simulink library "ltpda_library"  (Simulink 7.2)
settings: Solver=ode45  SolverMode=SingleTasking  StartTime=0.0  StopTime=10.0  RelTol=1e-3
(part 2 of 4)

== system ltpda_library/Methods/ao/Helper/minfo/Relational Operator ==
  eq : Subsystem  Tag=method minfo  AncestorBlock=libraryBase/function
  ne : Subsystem  Tag=method minfo  AncestorBlock=libraryBase/function

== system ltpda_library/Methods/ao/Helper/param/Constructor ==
  param : Subsystem  Tag=method param  AncestorBlock=libraryBase/constructor

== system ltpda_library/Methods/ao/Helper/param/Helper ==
  isprop : Subsystem  Tag=method param  AncestorBlock=libraryBase/function
  mux : Subsystem  Tag=method param  AncestorBlock=libraryBase/function

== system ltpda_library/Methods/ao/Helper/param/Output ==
  char : Subsystem  Tag=method param  AncestorBlock=libraryBase/output
  display : Subsystem  Tag=method param  AncestorBlock=libraryBase/output
  string : Subsystem  Tag=method param  AncestorBlock=libraryBase/output

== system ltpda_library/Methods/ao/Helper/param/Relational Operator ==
  eq : Subsystem  Tag=method param  AncestorBlock=libraryBase/function
  ne : Subsystem  Tag=method param  AncestorBlock=libraryBase/function

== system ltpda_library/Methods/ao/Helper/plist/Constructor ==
  plist : Subsystem  Tag=method plist  AncestorBlock=libraryBase/constructor
  rebuild : Subsystem  Tag=method parfrac  AncestorBlock=libraryBase/constructor

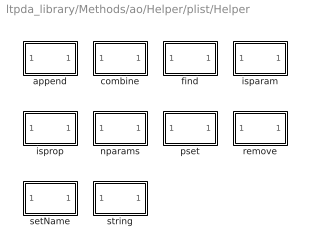
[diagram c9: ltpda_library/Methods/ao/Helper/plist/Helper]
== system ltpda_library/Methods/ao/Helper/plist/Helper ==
  append : Subsystem  Tag=method plist  AncestorBlock=libraryBase/function
  combine : Subsystem  Tag=method plist  AncestorBlock=libraryBase/function
  find : Subsystem  Tag=method plist  AncestorBlock=libraryBase/function
  isparam : Subsystem  Tag=method plist  AncestorBlock=libraryBase/function
  isprop : Subsystem  Tag=method plist  AncestorBlock=libraryBase/function
  nparams : Subsystem  Tag=method plist  AncestorBlock=libraryBase/function
  pset : Subsystem  Tag=method plist  AncestorBlock=libraryBase/function
  remove : Subsystem  Tag=method plist  AncestorBlock=libraryBase/function
  setName : Subsystem  Tag=method plist  AncestorBlock=libraryBase/function
  string : Subsystem  Tag=method plist  AncestorBlock=libraryBase/function

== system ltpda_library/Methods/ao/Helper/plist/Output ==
  char : Subsystem  Tag=method plist  AncestorBlock=libraryBase/output
  display : Subsystem  Tag=method plist  AncestorBlock=libraryBase/output
  save : Subsystem  Tag=method plist  AncestorBlock=libraryBase/output

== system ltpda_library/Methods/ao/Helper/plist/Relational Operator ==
  eq : Subsystem  Tag=method plist  AncestorBlock=libraryBase/function
  ne : Subsystem  Tag=method plist  AncestorBlock=libraryBase/function

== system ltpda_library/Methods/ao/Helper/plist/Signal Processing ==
  resp : Subsystem  Tag=method plist  AncestorBlock=libraryBase/function

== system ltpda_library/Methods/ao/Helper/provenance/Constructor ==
  provenance : Subsystem  Tag=method provenance  AncestorBlock=libraryBase/constructor

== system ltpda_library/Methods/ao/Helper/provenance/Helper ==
  isprop : Subsystem  Tag=method provenance  AncestorBlock=libraryBase/function

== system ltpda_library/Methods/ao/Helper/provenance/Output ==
  char : Subsystem  Tag=method provenance  AncestorBlock=libraryBase/output
  display : Subsystem  Tag=method provenance  AncestorBlock=libraryBase/output
  string : Subsystem  Tag=method provenance  AncestorBlock=libraryBase/output

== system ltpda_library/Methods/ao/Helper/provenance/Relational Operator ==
  eq : Subsystem  Tag=method provenance  AncestorBlock=libraryBase/function
  ne : Subsystem  Tag=method provenance  AncestorBlock=libraryBase/function

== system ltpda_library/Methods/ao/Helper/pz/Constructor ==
  pz : Subsystem  Tag=method pz  AncestorBlock=libraryBase/constructor

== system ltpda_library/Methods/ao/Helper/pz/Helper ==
  isprop : Subsystem  Tag=method pz  AncestorBlock=libraryBase/function

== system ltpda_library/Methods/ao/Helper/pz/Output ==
  char : Subsystem  Tag=method pz  AncestorBlock=libraryBase/output
  display : Subsystem  Tag=method pz  AncestorBlock=libraryBase/output
  string : Subsystem  Tag=method pz  AncestorBlock=libraryBase/output

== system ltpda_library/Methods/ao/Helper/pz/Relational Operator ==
  eq : Subsystem  Tag=method pz  AncestorBlock=libraryBase/function
  ne : Subsystem  Tag=method pz  AncestorBlock=libraryBase/function

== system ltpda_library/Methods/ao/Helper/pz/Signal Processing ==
  resp : Subsystem  Tag=method pz  AncestorBlock=libraryBase/function

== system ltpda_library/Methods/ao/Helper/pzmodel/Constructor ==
  pzmodel : Subsystem  Tag=method pzmodel  AncestorBlock=libraryBase/constructor
  rebuild : Subsystem  Tag=method pzmodel  AncestorBlock=libraryBase/constructor

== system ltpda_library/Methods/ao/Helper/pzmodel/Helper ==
  isprop : Subsystem  Tag=method pzmodel  AncestorBlock=libraryBase/function
  setIunits : Subsystem  Tag=method pzmodel  AncestorBlock=libraryBase/function
  setName : Subsystem  Tag=method pzmodel  AncestorBlock=libraryBase/function
  setOunits : Subsystem  Tag=method pzmodel  AncestorBlock=libraryBase/function
  setProperties : Subsystem  Tag=method pzmodel  AncestorBlock=libraryBase/function
  string : Subsystem  Tag=method pzmodel  AncestorBlock=libraryBase/function

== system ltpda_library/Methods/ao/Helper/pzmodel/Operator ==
  tomfir : Subsystem  Tag=method pzmodel  AncestorBlock=libraryBase/function
  tomiir : Subsystem  Tag=method pzmodel  AncestorBlock=libraryBase/function

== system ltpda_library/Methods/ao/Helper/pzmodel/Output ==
  char : Subsystem  Tag=method pzmodel  AncestorBlock=libraryBase/output
  display : Subsystem  Tag=method pzmodel  AncestorBlock=libraryBase/output
  save : Subsystem  Tag=method pzmodel  AncestorBlock=libraryBase/output
  type : Subsystem  Tag=method pzmodel  AncestorBlock=libraryBase/output

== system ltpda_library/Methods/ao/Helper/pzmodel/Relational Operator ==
  eq : Subsystem  Tag=method pzmodel  AncestorBlock=libraryBase/function
  ne : Subsystem  Tag=method pzmodel  AncestorBlock=libraryBase/function

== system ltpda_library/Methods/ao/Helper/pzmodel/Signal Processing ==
  fngen : Subsystem  Tag=method pzmodel  AncestorBlock=libraryBase/function
  resp : Subsystem  Tag=method pzmodel  AncestorBlock=libraryBase/function

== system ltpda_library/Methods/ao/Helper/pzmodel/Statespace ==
  report : Subsystem  Tag=method pzmodel  AncestorBlock=libraryBase/function

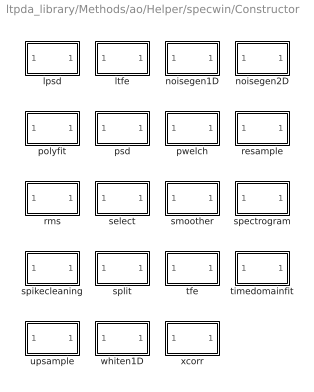
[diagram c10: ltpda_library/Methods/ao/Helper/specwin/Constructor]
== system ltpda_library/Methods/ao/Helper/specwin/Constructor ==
  lpsd : Subsystem  Tag=method specwin  AncestorBlock=libraryBase/constructor  Tag=method ao  AncestorBlock=libraryBase/function
  ltfe : Subsystem  Tag=method ao  AncestorBlock=libraryBase/function
  noisegen1D : Subsystem  Tag=method ao  AncestorBlock=libraryBase/function
  noisegen2D : Subsystem  Tag=method ao  AncestorBlock=libraryBase/function
  polyfit : Subsystem  Tag=method ao  AncestorBlock=libraryBase/function
  psd : Subsystem  Tag=method ao  AncestorBlock=libraryBase/function
  pwelch : Subsystem  Tag=method ao  AncestorBlock=libraryBase/function
  resample : Subsystem  Tag=method ao  AncestorBlock=libraryBase/function
  rms : Subsystem  Tag=method ao  AncestorBlock=libraryBase/function
  select : Subsystem  Tag=method ao  AncestorBlock=libraryBase/function
  smoother : Subsystem  Tag=method ao  AncestorBlock=libraryBase/function
  spectrogram : Subsystem  Tag=method ao  AncestorBlock=libraryBase/function
  spikecleaning : Subsystem  Tag=method ao  AncestorBlock=libraryBase/function
  split : Subsystem  Tag=method ao  AncestorBlock=libraryBase/function
  tfe : Subsystem  Tag=method ao  AncestorBlock=libraryBase/function
  timedomainfit : Subsystem  Tag=method ao  AncestorBlock=libraryBase/function
  upsample : Subsystem  Tag=method ao  AncestorBlock=libraryBase/function
  whiten1D : Subsystem  Tag=method ao  AncestorBlock=libraryBase/function
  xcorr : Subsystem  Tag=method ao  AncestorBlock=libraryBase/function

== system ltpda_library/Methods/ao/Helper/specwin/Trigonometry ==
  acos : Subsystem  Tag=method ao  AncestorBlock=libraryBase/function
  asin : Subsystem  Tag=method ao  AncestorBlock=libraryBase/function
  atan : Subsystem  Tag=method ao  AncestorBlock=libraryBase/function
  atan2 : Subsystem  Tag=method ao  AncestorBlock=libraryBase/function
  cos : Subsystem  Tag=method ao  AncestorBlock=libraryBase/function
  sin : Subsystem  Tag=method ao  AncestorBlock=libraryBase/function
  tan : Subsystem  Tag=method ao  AncestorBlock=libraryBase/function

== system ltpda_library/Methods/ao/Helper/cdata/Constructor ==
  cdata : Subsystem  Tag=method cdata  AncestorBlock=libraryBase/constructor

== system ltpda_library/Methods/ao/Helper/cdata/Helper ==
  isprop : Subsystem  Tag=method cdata  AncestorBlock=libraryBase/function

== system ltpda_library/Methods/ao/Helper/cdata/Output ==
  display : Subsystem  Tag=method cdata  AncestorBlock=libraryBase/output

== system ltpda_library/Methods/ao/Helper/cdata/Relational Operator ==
  eq : Subsystem  Tag=method cdata  AncestorBlock=libraryBase/function
  ne : Subsystem  Tag=method cdata  AncestorBlock=libraryBase/function

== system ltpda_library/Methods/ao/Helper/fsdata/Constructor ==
  fsdata : Subsystem  Tag=method fsdata  AncestorBlock=libraryBase/constructor

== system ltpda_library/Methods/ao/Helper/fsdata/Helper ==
  isprop : Subsystem  Tag=method fsdata  AncestorBlock=libraryBase/function

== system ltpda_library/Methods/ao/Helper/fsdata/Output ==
  char : Subsystem  Tag=method fsdata  AncestorBlock=libraryBase/output
  display : Subsystem  Tag=method fsdata  AncestorBlock=libraryBase/output

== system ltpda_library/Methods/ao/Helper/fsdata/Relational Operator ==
  eq : Subsystem  Tag=method fsdata  AncestorBlock=libraryBase/function
  ne : Subsystem  Tag=method fsdata  AncestorBlock=libraryBase/function

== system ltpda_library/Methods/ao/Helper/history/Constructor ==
  history : Subsystem  Tag=method history  AncestorBlock=libraryBase/constructor
  rebuild : Subsystem  Tag=method history  AncestorBlock=libraryBase/constructor

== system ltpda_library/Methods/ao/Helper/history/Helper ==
  isprop : Subsystem  Tag=method history  AncestorBlock=libraryBase/function

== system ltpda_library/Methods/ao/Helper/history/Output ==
  char : Subsystem  Tag=method history  AncestorBlock=libraryBase/output
  display : Subsystem  Tag=method history  AncestorBlock=libraryBase/output
  dotview : Subsystem  Tag=method history  AncestorBlock=libraryBase/output
  hist2dot : Subsystem  Tag=method history  AncestorBlock=libraryBase/output
  hist2m : Subsystem  Tag=method history  AncestorBlock=libraryBase/output
  plot : Subsystem  Tag=method history  AncestorBlock=libraryBase/output
  string : Subsystem  Tag=method history  AncestorBlock=libraryBase/output

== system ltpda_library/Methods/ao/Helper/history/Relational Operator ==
  eq : Subsystem  Tag=method history  AncestorBlock=libraryBase/function
  ne : Subsystem  Tag=method history  AncestorBlock=libraryBase/function

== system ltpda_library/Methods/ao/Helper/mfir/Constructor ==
  mfir : Subsystem  Tag=method mfir  AncestorBlock=libraryBase/constructor
  rebuild : Subsystem  Tag=method mfir  AncestorBlock=libraryBase/constructor

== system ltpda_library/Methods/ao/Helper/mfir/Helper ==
  isprop : Subsystem  Tag=method mfir  AncestorBlock=libraryBase/function
  redesign : Subsystem  Tag=method mfir  AncestorBlock=libraryBase/function
  setIunits : Subsystem  Tag=method mfir  AncestorBlock=libraryBase/function
  setName : Subsystem  Tag=method mfir  AncestorBlock=libraryBase/function
  setOunits : Subsystem  Tag=method mfir  AncestorBlock=libraryBase/function
  setProperties : Subsystem  Tag=method mfir  AncestorBlock=libraryBase/function

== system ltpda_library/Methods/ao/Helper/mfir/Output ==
  char : Subsystem  Tag=method mfir  AncestorBlock=libraryBase/output
  display : Subsystem  Tag=method mfir  AncestorBlock=libraryBase/output
  report : Subsystem  Tag=method mfir  AncestorBlock=libraryBase/output
  save : Subsystem  Tag=method mfir  AncestorBlock=libraryBase/output
  string : Subsystem  Tag=method mfir  AncestorBlock=libraryBase/output
  type : Subsystem  Tag=method mfir  AncestorBlock=libraryBase/output

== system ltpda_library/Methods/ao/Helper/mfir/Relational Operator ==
  eq : Subsystem  Tag=method mfir  AncestorBlock=libraryBase/function
  ne : Subsystem  Tag=method mfir  AncestorBlock=libraryBase/function

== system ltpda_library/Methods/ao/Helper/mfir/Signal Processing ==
  oldresp : Subsystem  Tag=method mfir  AncestorBlock=libraryBase/function
  resp : Subsystem  Tag=method mfir  AncestorBlock=libraryBase/function

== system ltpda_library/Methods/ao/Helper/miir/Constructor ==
  miir : Subsystem  Tag=method miir  AncestorBlock=libraryBase/constructor
  rebuild : Subsystem  Tag=method miir  AncestorBlock=libraryBase/constructor

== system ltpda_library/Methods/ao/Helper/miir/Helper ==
  isprop : Subsystem  Tag=method miir  AncestorBlock=libraryBase/function
  redesign : Subsystem  Tag=method miir  AncestorBlock=libraryBase/function
  setIunits : Subsystem  Tag=method miir  AncestorBlock=libraryBase/function
  setName : Subsystem  Tag=method miir  AncestorBlock=libraryBase/function
  setOunits : Subsystem  Tag=method miir  AncestorBlock=libraryBase/function
  setProperties : Subsystem  Tag=method miir  AncestorBlock=libraryBase/function

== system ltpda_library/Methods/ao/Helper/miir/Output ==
  char : Subsystem  Tag=method miir  AncestorBlock=libraryBase/output
  display : Subsystem  Tag=method miir  AncestorBlock=libraryBase/output
  report : Subsystem  Tag=method miir  AncestorBlock=libraryBase/output
  save : Subsystem  Tag=method miir  AncestorBlock=libraryBase/output
  string : Subsystem  Tag=method miir  AncestorBlock=libraryBase/output
  type : Subsystem  Tag=method miir  AncestorBlock=libraryBase/output

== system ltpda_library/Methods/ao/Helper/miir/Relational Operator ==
  eq : Subsystem  Tag=method miir  AncestorBlock=libraryBase/function
  ne : Subsystem  Tag=method miir  AncestorBlock=libraryBase/function

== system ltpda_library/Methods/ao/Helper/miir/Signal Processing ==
  oldresp : Subsystem  Tag=method miir  AncestorBlock=libraryBase/function
  resp : Subsystem  Tag=method miir  AncestorBlock=libraryBase/function

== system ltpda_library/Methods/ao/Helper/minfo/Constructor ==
  minfo : Subsystem  Tag=method minfo  AncestorBlock=libraryBase/constructor

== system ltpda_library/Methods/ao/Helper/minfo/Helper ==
  isprop : Subsystem  Tag=method minfo  AncestorBlock=libraryBase/function

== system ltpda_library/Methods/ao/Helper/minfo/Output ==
  char : Subsystem  Tag=method minfo  AncestorBlock=libraryBase/output
  display : Subsystem  Tag=method minfo  AncestorBlock=libraryBase/output

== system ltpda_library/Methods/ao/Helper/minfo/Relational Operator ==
  eq : Subsystem  Tag=method minfo  AncestorBlock=libraryBase/function
  ne : Subsystem  Tag=method minfo  AncestorBlock=libraryBase/function

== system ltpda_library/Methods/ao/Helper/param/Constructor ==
  param : Subsystem  Tag=method param  AncestorBlock=libraryBase/constructor

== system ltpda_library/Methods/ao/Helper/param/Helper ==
  isprop : Subsystem  Tag=method param  AncestorBlock=libraryBase/function
  mux : Subsystem  Tag=method param  AncestorBlock=libraryBase/function

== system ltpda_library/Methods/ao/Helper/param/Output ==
  char : Subsystem  Tag=method param  AncestorBlock=libraryBase/output
  display : Subsystem  Tag=method param  AncestorBlock=libraryBase/output
  string : Subsystem  Tag=method param  AncestorBlock=libraryBase/output

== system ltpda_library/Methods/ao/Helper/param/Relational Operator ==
  eq : Subsystem  Tag=method param  AncestorBlock=libraryBase/function
  ne : Subsystem  Tag=method param  AncestorBlock=libraryBase/function

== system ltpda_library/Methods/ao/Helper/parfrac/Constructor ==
  parfrac : Subsystem  Tag=method parfrac  AncestorBlock=libraryBase/constructor
  rebuild : Subsystem  Tag=method parfrac  AncestorBlock=libraryBase/constructor

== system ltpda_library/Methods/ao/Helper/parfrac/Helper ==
  isprop : Subsystem  Tag=method parfrac  AncestorBlock=libraryBase/function
  setIunits : Subsystem  Tag=method parfrac  AncestorBlock=libraryBase/function
  setName : Subsystem  Tag=method parfrac  AncestorBlock=libraryBase/function
  setOunits : Subsystem  Tag=method parfrac  AncestorBlock=libraryBase/function
  setProperties : Subsystem  Tag=method parfrac  AncestorBlock=libraryBase/function
  string : Subsystem  Tag=method parfrac  AncestorBlock=libraryBase/function

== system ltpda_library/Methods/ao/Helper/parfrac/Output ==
  char : Subsystem  Tag=method parfrac  AncestorBlock=libraryBase/output
  display : Subsystem  Tag=method parfrac  AncestorBlock=libraryBase/output
  report : Subsystem  Tag=method parfrac  AncestorBlock=libraryBase/output
  save : Subsystem  Tag=method parfrac  AncestorBlock=libraryBase/output
  type : Subsystem  Tag=method parfrac  AncestorBlock=libraryBase/output

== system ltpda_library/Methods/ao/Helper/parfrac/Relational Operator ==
  eq : Subsystem  Tag=method parfrac  AncestorBlock=libraryBase/function
  ne : Subsystem  Tag=method parfrac  AncestorBlock=libraryBase/function

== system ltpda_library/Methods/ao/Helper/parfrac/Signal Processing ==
  resp : Subsystem  Tag=method parfrac  AncestorBlock=libraryBase/function

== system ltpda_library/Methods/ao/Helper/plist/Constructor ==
  plist : Subsystem  Tag=method plist  AncestorBlock=libraryBase/constructor

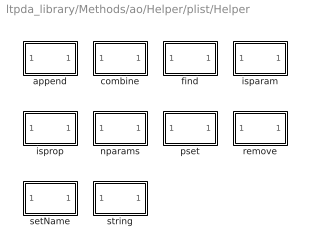
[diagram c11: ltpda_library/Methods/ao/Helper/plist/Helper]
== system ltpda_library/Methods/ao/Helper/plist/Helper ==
  append : Subsystem  Tag=method plist  AncestorBlock=libraryBase/function
  combine : Subsystem  Tag=method plist  AncestorBlock=libraryBase/function
  find : Subsystem  Tag=method plist  AncestorBlock=libraryBase/function
  isparam : Subsystem  Tag=method plist  AncestorBlock=libraryBase/function
  isprop : Subsystem  Tag=method plist  AncestorBlock=libraryBase/function
  nparams : Subsystem  Tag=method plist  AncestorBlock=libraryBase/function
  pset : Subsystem  Tag=method plist  AncestorBlock=libraryBase/function
  remove : Subsystem  Tag=method plist  AncestorBlock=libraryBase/function
  setName : Subsystem  Tag=method plist  AncestorBlock=libraryBase/function
  string : Subsystem  Tag=method plist  AncestorBlock=libraryBase/function

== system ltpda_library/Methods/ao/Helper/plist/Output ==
  char : Subsystem  Tag=method plist  AncestorBlock=libraryBase/output
  display : Subsystem  Tag=method plist  AncestorBlock=libraryBase/output
  save : Subsystem  Tag=method plist  AncestorBlock=libraryBase/output

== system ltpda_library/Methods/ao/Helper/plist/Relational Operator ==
  eq : Subsystem  Tag=method plist  AncestorBlock=libraryBase/function
  ne : Subsystem  Tag=method plist  AncestorBlock=libraryBase/function

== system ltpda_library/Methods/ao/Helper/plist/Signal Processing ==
  resp : Subsystem  Tag=method plist  AncestorBlock=libraryBase/function

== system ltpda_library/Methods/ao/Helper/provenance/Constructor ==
  provenance : Subsystem  Tag=method provenance  AncestorBlock=libraryBase/constructor

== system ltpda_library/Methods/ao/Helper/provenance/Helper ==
  isprop : Subsystem  Tag=method provenance  AncestorBlock=libraryBase/function

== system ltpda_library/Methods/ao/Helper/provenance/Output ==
  char : Subsystem  Tag=method provenance  AncestorBlock=libraryBase/output
  display : Subsystem  Tag=method provenance  AncestorBlock=libraryBase/output
  string : Subsystem  Tag=method provenance  AncestorBlock=libraryBase/output

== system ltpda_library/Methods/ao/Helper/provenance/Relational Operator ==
  eq : Subsystem  Tag=method provenance  AncestorBlock=libraryBase/function
  ne : Subsystem  Tag=method provenance  AncestorBlock=libraryBase/function

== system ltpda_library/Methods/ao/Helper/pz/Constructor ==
  pz : Subsystem  Tag=method pz  AncestorBlock=libraryBase/constructor

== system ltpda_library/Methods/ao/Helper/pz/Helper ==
  isprop : Subsystem  Tag=method pz  AncestorBlock=libraryBase/function

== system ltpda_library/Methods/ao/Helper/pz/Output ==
  char : Subsystem  Tag=method pz  AncestorBlock=libraryBase/output
  display : Subsystem  Tag=method pz  AncestorBlock=libraryBase/output
  string : Subsystem  Tag=method pz  AncestorBlock=libraryBase/output

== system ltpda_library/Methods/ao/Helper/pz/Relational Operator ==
  eq : Subsystem  Tag=method pz  AncestorBlock=libraryBase/function
  ne : Subsystem  Tag=method pz  AncestorBlock=libraryBase/function

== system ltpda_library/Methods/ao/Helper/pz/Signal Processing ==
  resp : Subsystem  Tag=method pz  AncestorBlock=libraryBase/function

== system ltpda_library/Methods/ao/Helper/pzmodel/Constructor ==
  pzmodel : Subsystem  Tag=method pzmodel  AncestorBlock=libraryBase/constructor
  rebuild : Subsystem  Tag=method pzmodel  AncestorBlock=libraryBase/constructor

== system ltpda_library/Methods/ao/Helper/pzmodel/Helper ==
  isprop : Subsystem  Tag=method pzmodel  AncestorBlock=libraryBase/function
  setIunits : Subsystem  Tag=method pzmodel  AncestorBlock=libraryBase/function
  setName : Subsystem  Tag=method pzmodel  AncestorBlock=libraryBase/function
  setOunits : Subsystem  Tag=method pzmodel  AncestorBlock=libraryBase/function
  setProperties : Subsystem  Tag=method pzmodel  AncestorBlock=libraryBase/function
  string : Subsystem  Tag=method pzmodel  AncestorBlock=libraryBase/function

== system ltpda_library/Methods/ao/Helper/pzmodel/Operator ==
  tomfir : Subsystem  Tag=method pzmodel  AncestorBlock=libraryBase/function
  tomiir : Subsystem  Tag=method pzmodel  AncestorBlock=libraryBase/function

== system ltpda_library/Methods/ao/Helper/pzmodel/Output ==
  char : Subsystem  Tag=method pzmodel  AncestorBlock=libraryBase/output
  display : Subsystem  Tag=method pzmodel  AncestorBlock=libraryBase/output
  report : Subsystem  Tag=method pzmodel  AncestorBlock=libraryBase/output
  save : Subsystem  Tag=method pzmodel  AncestorBlock=libraryBase/output
  type : Subsystem  Tag=method pzmodel  AncestorBlock=libraryBase/output

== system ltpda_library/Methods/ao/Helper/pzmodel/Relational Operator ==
  eq : Subsystem  Tag=method pzmodel  AncestorBlock=libraryBase/function
  ne : Subsystem  Tag=method pzmodel  AncestorBlock=libraryBase/function

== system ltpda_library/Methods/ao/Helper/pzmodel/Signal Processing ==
  fngen : Subsystem  Tag=method pzmodel  AncestorBlock=libraryBase/function
  resp : Subsystem  Tag=method pzmodel  AncestorBlock=libraryBase/function

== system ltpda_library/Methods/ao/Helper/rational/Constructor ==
  rational : Subsystem  Tag=method rational  AncestorBlock=libraryBase/constructor
  rebuild : Subsystem  Tag=method rational  AncestorBlock=libraryBase/constructor

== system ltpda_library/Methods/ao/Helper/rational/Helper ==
  isprop : Subsystem  Tag=method rational  AncestorBlock=libraryBase/function
  setIunits : Subsystem  Tag=method rational  AncestorBlock=libraryBase/function
  setName : Subsystem  Tag=method rational  AncestorBlock=libraryBase/function
  setOunits : Subsystem  Tag=method rational  AncestorBlock=libraryBase/function
  setProperties : Subsystem  Tag=method rational  AncestorBlock=libraryBase/function
  string : Subsystem  Tag=method rational  AncestorBlock=libraryBase/function

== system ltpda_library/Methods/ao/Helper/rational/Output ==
  char : Subsystem  Tag=method rational  AncestorBlock=libraryBase/output
  display : Subsystem  Tag=method rational  AncestorBlock=libraryBase/output
  report : Subsystem  Tag=method rational  AncestorBlock=libraryBase/output
  save : Subsystem  Tag=method rational  AncestorBlock=libraryBase/output
  type : Subsystem  Tag=method rational  AncestorBlock=libraryBase/output

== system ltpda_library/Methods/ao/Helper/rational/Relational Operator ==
  eq : Subsystem  Tag=method rational  AncestorBlock=libraryBase/function
  ne : Subsystem  Tag=method rational  AncestorBlock=libraryBase/function

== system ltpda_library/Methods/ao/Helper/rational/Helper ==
  isprop : Subsystem  Tag=method specwin  AncestorBlock=libraryBase/function

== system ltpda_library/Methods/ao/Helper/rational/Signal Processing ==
  resp : Subsystem  Tag=method specwin  Tag=method rational  AncestorBlock=libraryBase/output  AncestorBlock=libraryBase/function

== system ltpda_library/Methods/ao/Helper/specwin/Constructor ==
  specwin : Subsystem  Tag=method specwin  AncestorBlock=libraryBase/constructor

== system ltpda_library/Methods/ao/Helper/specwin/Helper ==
  isprop : Subsystem  Tag=method specwin  AncestorBlock=libraryBase/output  Tag=method specwin  AncestorBlock=libraryBase/function
  char : Subsystem  Tag=method specwin  Tag=method specwin  AncestorBlock=libraryBase/output
  display : Subsystem  Tag=method specwin  AncestorBlock=libraryBase/output
  plot : Subsystem  Tag=method specwin  AncestorBlock=libraryBase/output  Tag=method specwin  AncestorBlock=libraryBase/output
  string : Subsystem  Tag=method specwin  AncestorBlock=libraryBase/output

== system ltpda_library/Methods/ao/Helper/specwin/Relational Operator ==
  eq : Subsystem  Tag=method specwin  AncestorBlock=libraryBase/function  AncestorBlock=libraryBase/function
  ne : Subsystem  Tag=method specwin  AncestorBlock=libraryBase/function  AncestorBlock=libraryBase/function

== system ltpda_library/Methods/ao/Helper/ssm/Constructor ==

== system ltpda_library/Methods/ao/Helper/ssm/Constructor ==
  rebuild : Subsystem  Tag=method ssm  AncestorBlock=libraryBase/constructor  Tag=method ssm  AncestorBlock=libraryBase/constructor
  ssm : Subsystem  Tag=method ssm  AncestorBlock=libraryBase/constructor  Tag=method ssm  AncestorBlock=libraryBase/constructor

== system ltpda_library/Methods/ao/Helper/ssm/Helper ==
  findParams : Subsystem  Tag=method ssm  AncestorBlock=libraryBase/function  Tag=method ssm  AncestorBlock=libraryBase/function
  isprop : Subsystem  Tag=method ssm  AncestorBlock=libraryBase/function  Tag=method ssm  AncestorBlock=libraryBase/function
  setName : Subsystem  Tag=method ssm  AncestorBlock=libraryBase/function

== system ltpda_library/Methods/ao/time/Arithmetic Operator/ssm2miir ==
  In1 : Inport  OutDataType=sfix(16)  OutScaling=2^0
  ssm2miir : M-S-Function  Tag=ssm2miir  FunctionName=ltpdasim
  Out1 : Outport  OutDataType=sfix(16)  OutScaling=2^0
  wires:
  In1/1 -> ssm2miir/1
  ssm2miir/1 -> Out1/1

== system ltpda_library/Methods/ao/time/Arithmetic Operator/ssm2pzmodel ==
  In1 : Inport  OutDataType=sfix(16)  OutScaling=2^0
  ssm2pzmodel : M-S-Function  Tag=ssm2pzmodel  FunctionName=ltpdasim
  Out1 : Outport  OutDataType=sfix(16)  OutScaling=2^0
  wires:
  In1/1 -> ssm2pzmodel/1
  ssm2pzmodel/1 -> Out1/1

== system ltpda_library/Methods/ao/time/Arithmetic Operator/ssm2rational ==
  In1 : Inport  OutDataType=sfix(16)  OutScaling=2^0
  ssm2rational : M-S-Function  Tag=ssm2rational  FunctionName=ltpdasim
  Out1 : Outport  OutDataType=sfix(16)  OutScaling=2^0
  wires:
  In1/1 -> ssm2rational/1
  ssm2rational/1 -> Out1/1

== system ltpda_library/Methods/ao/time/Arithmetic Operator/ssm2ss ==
  In1 : Inport  OutDataType=sfix(16)  OutScaling=2^0
  ssm2ss : M-S-Function  Tag=ssm2ss  FunctionName=ltpdasim
  Out1 : Outport  OutDataType=sfix(16)  OutScaling=2^0
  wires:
  In1/1 -> ssm2ss/1
  ssm2ss/1 -> Out1/1

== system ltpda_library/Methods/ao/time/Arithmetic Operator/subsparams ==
  In1 : Inport  OutDataType=sfix(16)  OutScaling=2^0
  subsparams : M-S-Function  Tag=subsparams  FunctionName=ltpdasim
  Out1 : Outport  OutDataType=sfix(16)  OutScaling=2^0
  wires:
  In1/1 -> subsparams/1
  subsparams/1 -> Out1/1

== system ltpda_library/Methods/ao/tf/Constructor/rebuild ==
  Ground : Ground
  rebuild : M-S-Function  Tag=rebuild  FunctionName=ltpdasim
  Out1 : Outport  OutDataType=sfix(16)  OutScaling=2^0
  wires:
  Ground/1 -> rebuild/1
  rebuild/1 -> Out1/1

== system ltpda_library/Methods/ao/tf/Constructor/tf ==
  Ground : Ground
  tf : M-S-Function  Tag=tf  FunctionName=ltpdasim
  Out1 : Outport  OutDataType=sfix(16)  OutScaling=2^0
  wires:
  Ground/1 -> tf/1
  tf/1 -> Out1/1

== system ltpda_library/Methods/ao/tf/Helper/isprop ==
  In1 : Inport  OutDataType=sfix(16)  OutScaling=2^0
  isprop : M-S-Function  Tag=isprop  FunctionName=ltpdasim
  Out1 : Outport  OutDataType=sfix(16)  OutScaling=2^0
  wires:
  In1/1 -> isprop/1
  isprop/1 -> Out1/1

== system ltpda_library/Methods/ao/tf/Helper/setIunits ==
  In1 : Inport  OutDataType=sfix(16)  OutScaling=2^0
  setIunits : M-S-Function  Tag=setIunits  FunctionName=ltpdasim
  Out1 : Outport  OutDataType=sfix(16)  OutScaling=2^0
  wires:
  In1/1 -> setIunits/1
  setIunits/1 -> Out1/1

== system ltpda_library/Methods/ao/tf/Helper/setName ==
  In1 : Inport  OutDataType=sfix(16)  OutScaling=2^0
  setName : M-S-Function  Tag=setName  FunctionName=ltpdasim
  Out1 : Outport  OutDataType=sfix(16)  OutScaling=2^0
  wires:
  In1/1 -> setName/1
  setName/1 -> Out1/1

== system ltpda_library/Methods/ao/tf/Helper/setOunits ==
  In1 : Inport  OutDataType=sfix(16)  OutScaling=2^0
  setOunits : M-S-Function  Tag=setOunits  FunctionName=ltpdasim
  Out1 : Outport  OutDataType=sfix(16)  OutScaling=2^0
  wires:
  In1/1 -> setOunits/1
  setOunits/1 -> Out1/1

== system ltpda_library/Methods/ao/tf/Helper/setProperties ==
  In1 : Inport  OutDataType=sfix(16)  OutScaling=2^0
  setProperties : M-S-Function  Tag=setProperties  FunctionName=ltpdasim
  Out1 : Outport  OutDataType=sfix(16)  OutScaling=2^0
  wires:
  In1/1 -> setProperties/1
  setProperties/1 -> Out1/1

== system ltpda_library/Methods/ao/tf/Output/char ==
  In1 : Inport  OutDataType=sfix(16)  OutScaling=2^0
  Terminator : Terminator
  char : M-S-Function  Tag=char  FunctionName=ltpdasim
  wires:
  char/1 -> Terminator/1
  In1/1 -> char/1

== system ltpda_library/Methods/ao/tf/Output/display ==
  In1 : Inport  OutDataType=sfix(16)  OutScaling=2^0
  Terminator : Terminator
  display : M-S-Function  Tag=display  FunctionName=ltpdasim
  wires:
  display/1 -> Terminator/1
  In1/1 -> display/1

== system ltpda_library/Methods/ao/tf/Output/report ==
  In1 : Inport  OutDataType=sfix(16)  OutScaling=2^0
  Terminator : Terminator
  report : M-S-Function  Tag=report  FunctionName=ltpdasim
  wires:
  report/1 -> Terminator/1
  In1/1 -> report/1

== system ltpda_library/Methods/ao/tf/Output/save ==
  In1 : Inport  OutDataType=sfix(16)  OutScaling=2^0
  Terminator : Terminator
  save : M-S-Function  Tag=save  FunctionName=ltpdasim
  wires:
  save/1 -> Terminator/1
  In1/1 -> save/1

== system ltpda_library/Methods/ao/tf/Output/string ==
  In1 : Inport  OutDataType=sfix(16)  OutScaling=2^0
  Terminator : Terminator
  string : M-S-Function  Tag=string  FunctionName=ltpdasim
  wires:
  string/1 -> Terminator/1
  In1/1 -> string/1

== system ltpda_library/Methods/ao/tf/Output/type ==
  In1 : Inport  OutDataType=sfix(16)  OutScaling=2^0
  Terminator : Terminator
  type : M-S-Function  Tag=type  FunctionName=ltpdasim
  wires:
  type/1 -> Terminator/1
  In1/1 -> type/1

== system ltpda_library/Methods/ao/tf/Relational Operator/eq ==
  In1 : Inport  OutDataType=sfix(16)  OutScaling=2^0
  eq : M-S-Function  Tag=eq  FunctionName=ltpdasim
  Out1 : Outport  OutDataType=sfix(16)  OutScaling=2^0
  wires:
  In1/1 -> eq/1
  eq/1 -> Out1/1

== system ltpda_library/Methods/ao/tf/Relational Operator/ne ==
  In1 : Inport  OutDataType=sfix(16)  OutScaling=2^0
  ne : M-S-Function  Tag=ne  FunctionName=ltpdasim
  Out1 : Outport  OutDataType=sfix(16)  OutScaling=2^0
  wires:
  In1/1 -> ne/1
  ne/1 -> Out1/1

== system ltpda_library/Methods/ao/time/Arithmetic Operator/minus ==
  In1 : Inport  OutDataType=sfix(16)  OutScaling=2^0
  minus : M-S-Function  Tag=minus  FunctionName=ltpdasim
  Out1 : Outport  OutDataType=sfix(16)  OutScaling=2^0
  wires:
  In1/1 -> minus/1
  minus/1 -> Out1/1

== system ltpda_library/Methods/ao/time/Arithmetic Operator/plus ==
  In1 : Inport  OutDataType=sfix(16)  OutScaling=2^0
  plus : M-S-Function  Tag=plus  FunctionName=ltpdasim
  Out1 : Outport  OutDataType=sfix(16)  OutScaling=2^0
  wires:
  In1/1 -> plus/1
  plus/1 -> Out1/1

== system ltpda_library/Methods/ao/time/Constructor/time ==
  Ground : Ground
  time : M-S-Function  Tag=time  FunctionName=ltpdasim
  Out1 : Outport  OutDataType=sfix(16)  OutScaling=2^0
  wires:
  Ground/1 -> time/1
  time/1 -> Out1/1

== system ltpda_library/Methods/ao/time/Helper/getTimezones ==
  In1 : Inport  OutDataType=sfix(16)  OutScaling=2^0
  getTimezones : M-S-Function  Tag=getTimezones  FunctionName=ltpdasim
  Out1 : Outport  OutDataType=sfix(16)  OutScaling=2^0
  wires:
  In1/1 -> getTimezones/1
  getTimezones/1 -> Out1/1

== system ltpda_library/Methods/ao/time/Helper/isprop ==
  In1 : Inport  OutDataType=sfix(16)  OutScaling=2^0
  isprop : M-S-Function  Tag=isprop  FunctionName=ltpdasim
  Out1 : Outport  OutDataType=sfix(16)  OutScaling=2^0
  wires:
  In1/1 -> isprop/1
  isprop/1 -> Out1/1

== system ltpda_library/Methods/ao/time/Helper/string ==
  In1 : Inport  OutDataType=sfix(16)  OutScaling=2^0
  string : M-S-Function  Tag=string  FunctionName=ltpdasim
  Out1 : Outport  OutDataType=sfix(16)  OutScaling=2^0
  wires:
  In1/1 -> string/1
  string/1 -> Out1/1

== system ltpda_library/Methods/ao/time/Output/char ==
  In1 : Inport  OutDataType=sfix(16)  OutScaling=2^0
  Terminator : Terminator
  char : M-S-Function  Tag=char  FunctionName=ltpdasim
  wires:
  char/1 -> Terminator/1
  In1/1 -> char/1

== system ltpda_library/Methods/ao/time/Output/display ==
  In1 : Inport  OutDataType=sfix(16)  OutScaling=2^0
  Terminator : Terminator
  display : M-S-Function  Tag=display  FunctionName=ltpdasim
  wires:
  display/1 -> Terminator/1
  In1/1 -> display/1

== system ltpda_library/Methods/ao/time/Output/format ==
  In1 : Inport  OutDataType=sfix(16)  OutScaling=2^0
  Terminator : Terminator
  format : M-S-Function  Tag=format  FunctionName=ltpdasim
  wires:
  format/1 -> Terminator/1
  In1/1 -> format/1

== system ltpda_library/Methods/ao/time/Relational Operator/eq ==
  In1 : Inport  OutDataType=sfix(16)  OutScaling=2^0
  eq : M-S-Function  Tag=eq  FunctionName=ltpdasim
  Out1 : Outport  OutDataType=sfix(16)  OutScaling=2^0
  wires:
  In1/1 -> eq/1
  eq/1 -> Out1/1

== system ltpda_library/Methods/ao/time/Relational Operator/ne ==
  In1 : Inport  OutDataType=sfix(16)  OutScaling=2^0
  format : M-S-Function  Tag=format  FunctionName=ltpdasim
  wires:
  format/1 -> ?Terminator/1
  In1/1 -> format/1

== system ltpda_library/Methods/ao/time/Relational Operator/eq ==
  In1 : Inport  OutDataType=sfix(16)  OutScaling=2^0
  eq : M-S-Function  Tag=eq  FunctionName=ltpdasim
  Out1 : Outport  OutDataType=sfix(16)  OutScaling=2^0
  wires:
  In1/1 -> eq/1
  eq/1 -> Out1/1

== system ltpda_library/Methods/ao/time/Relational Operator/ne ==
  In1 : Inport  OutDataType=sfix(16)  OutScaling=2^0
  ne : M-S-Function  Tag=ne  Tag=ne  FunctionName=ltpdasim
  Out1 : Outport  OutDataType=sfix(16)  OutScaling=2^0
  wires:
  In1/1 -> ne/1
  ne/1 -> Out1/1

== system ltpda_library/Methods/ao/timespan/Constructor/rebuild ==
  Ground : Ground
  rebuild : M-S-Function  Tag=rebuild  FunctionName=ltpdasim
  Out1 : Outport  OutDataType=sfix(16)  OutScaling=2^0
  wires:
  Ground/1 -> rebuild/1
  rebuild/1 -> Out1/1

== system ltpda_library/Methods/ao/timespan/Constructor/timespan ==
  Ground : Ground
  rebuild : M-S-Function  Tag=rebuild  FunctionName=ltpdasim
  Out1 : Outport  OutDataType=sfix(16)  OutScaling=2^0
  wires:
  Ground/1 -> rebuild/1
  rebuild/1 -> Out1/1

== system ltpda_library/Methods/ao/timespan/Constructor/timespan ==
  Ground : Ground
  timespan : M-S-Function  Tag=timespan  FunctionName=ltpdasim
  Out1 : Outport  OutDataType=sfix(16)  OutScaling=2^0
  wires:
  Ground/1 -> timespan/1
  timespan/1 -> Out1/1

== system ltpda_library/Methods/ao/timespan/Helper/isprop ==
  In1 : Inport  OutDataType=sfix(16)  OutScaling=2^0
  isprop : M-S-Function  Tag=isprop  FunctionName=ltpdasim
  Out1 : Outport  OutDataType=sfix(16)  OutScaling=2^0
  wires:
  In1/1 -> isprop/1
  isprop/1 -> Out1/1

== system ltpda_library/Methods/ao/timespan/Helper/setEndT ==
  In1 : Inport  OutDataType=sfix(16)  OutScaling=2^0
  setEndT : M-S-Function  Tag=setEndT  FunctionName=ltpdasim
  Out1 : Outport  OutDataType=sfix(16)  OutScaling=2^0
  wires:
  In1/1 -> setEndT/1
  setEndT/1 -> Out1/1

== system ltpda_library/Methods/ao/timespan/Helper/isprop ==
  In1 : Inport  OutDataType=sfix(16)  OutScaling=2^0
  isprop : M-S-Function  Tag=setName  Tag=isprop  FunctionName=ltpdasim
  Out1 : Outport  OutDataType=sfix(16)  OutScaling=2^0
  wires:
  In1/1 -> isprop/1
  isprop/1 -> Out1/1

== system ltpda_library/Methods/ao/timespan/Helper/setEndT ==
  In1 : Inport  OutDataType=sfix(16)  OutScaling=2^0
  setEndT : M-S-Function  Tag=setEndT  FunctionName=ltpdasim
  Out1 : Outport  OutDataType=sfix(16)  OutScaling=2^0
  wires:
  In1/1 -> setEndT/1
  setEndT/1 -> Out1/1

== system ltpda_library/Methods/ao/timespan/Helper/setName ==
  In1 : Inport  OutDataType=sfix(16)  OutScaling=2^0
  setName : M-S-Function  Tag=setProperties  Tag=setName  FunctionName=ltpdasim
  Out1 : Outport  OutDataType=sfix(16)  OutScaling=2^0
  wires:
  In1/1 -> setName/1
  setName/1 -> Out1/1

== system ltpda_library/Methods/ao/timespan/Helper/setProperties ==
  In1 : Inport  OutDataType=sfix(16)  OutScaling=2^0
  setProperties : M-S-Function  Tag=setStartT  Tag=setProperties  FunctionName=ltpdasim
  Out1 : Outport  OutDataType=sfix(16)  OutScaling=2^0
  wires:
  In1/1 -> setProperties/1
  setProperties/1 -> Out1/1

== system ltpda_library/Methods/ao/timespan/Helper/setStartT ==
  In1 : Inport  OutDataType=sfix(16)  OutScaling=2^0
  setStartT : M-S-Function  Tag=setTimeformat  Tag=setStartT  FunctionName=ltpdasim
  Out1 : Outport  OutDataType=sfix(16)  OutScaling=2^0
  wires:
  In1/1 -> setStartT/1
  setStartT/1 -> Out1/1

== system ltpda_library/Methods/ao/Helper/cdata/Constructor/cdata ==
  Ground : Ground
  cdata : M-S-Function  Tag=cdata  FunctionName=ltpdasim
  Out1 : Outport  OutDataType=sfix(16)  OutScaling=2^0
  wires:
  Ground/1 -> cdata/1
  cdata/1 -> Out1/1

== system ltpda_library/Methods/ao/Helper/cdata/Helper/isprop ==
  In1 : Inport  OutDataType=sfix(16)  OutScaling=2^0
  isprop : M-S-Function  Tag=isprop  FunctionName=ltpdasim
  Out1 : Outport  OutDataType=sfix(16)  OutScaling=2^0
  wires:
  In1/1 -> isprop/1
  isprop/1 -> Out1/1

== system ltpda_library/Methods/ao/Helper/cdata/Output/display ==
  In1 : Inport  OutDataType=sfix(16)  OutScaling=2^0
  Terminator : Terminator
  display : M-S-Function  Tag=display  FunctionName=ltpdasim
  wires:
  display/1 -> Terminator/1
  In1/1 -> display/1

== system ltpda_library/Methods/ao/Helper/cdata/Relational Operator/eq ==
  In1 : Inport  OutDataType=sfix(16)  OutScaling=2^0
  eq : M-S-Function  Tag=eq  FunctionName=ltpdasim
  Out1 : Outport  OutDataType=sfix(16)  OutScaling=2^0
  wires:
  In1/1 -> eq/1
  eq/1 -> Out1/1

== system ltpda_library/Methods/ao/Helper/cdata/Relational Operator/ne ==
  In1 : Inport  OutDataType=sfix(16)  OutScaling=2^0
  ne : M-S-Function  Tag=ne  FunctionName=ltpdasim
  Out1 : Outport  OutDataType=sfix(16)  OutScaling=2^0
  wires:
  In1/1 -> ne/1
  ne/1 -> Out1/1

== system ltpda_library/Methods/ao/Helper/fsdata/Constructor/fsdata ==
  Ground : Ground
  fsdata : M-S-Function  Tag=fsdata  FunctionName=ltpdasim
  Out1 : Outport  OutDataType=sfix(16)  OutScaling=2^0
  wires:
  Ground/1 -> fsdata/1
  fsdata/1 -> Out1/1

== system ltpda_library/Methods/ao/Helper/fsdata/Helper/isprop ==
  In1 : Inport  OutDataType=sfix(16)  OutScaling=2^0
  isprop : M-S-Function  Tag=isprop  FunctionName=ltpdasim
  Out1 : Outport  OutDataType=sfix(16)  OutScaling=2^0
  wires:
  In1/1 -> isprop/1
  isprop/1 -> Out1/1

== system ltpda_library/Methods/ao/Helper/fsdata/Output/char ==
  In1 : Inport  OutDataType=sfix(16)  OutScaling=2^0
  Terminator : Terminator
  char : M-S-Function  Tag=char  FunctionName=ltpdasim
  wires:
  char/1 -> Terminator/1
  In1/1 -> char/1

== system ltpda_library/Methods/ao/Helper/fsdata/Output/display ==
  In1 : Inport  OutDataType=sfix(16)  OutScaling=2^0
  Terminator : Terminator
  display : M-S-Function  Tag=display  FunctionName=ltpdasim
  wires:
  display/1 -> Terminator/1
  In1/1 -> display/1

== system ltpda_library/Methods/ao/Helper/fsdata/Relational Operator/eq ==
  In1 : Inport  OutDataType=sfix(16)  OutScaling=2^0
  eq : M-S-Function  Tag=eq  FunctionName=ltpdasim
  Out1 : Outport  OutDataType=sfix(16)  OutScaling=2^0
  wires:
  In1/1 -> eq/1
  eq/1 -> Out1/1

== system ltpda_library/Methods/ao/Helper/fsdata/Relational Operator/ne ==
  In1 : Inport  OutDataType=sfix(16)  OutScaling=2^0
  ne : M-S-Function  Tag=ne  FunctionName=ltpdasim
  Out1 : Outport  OutDataType=sfix(16)  OutScaling=2^0
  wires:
  In1/1 -> ne/1
  ne/1 -> Out1/1

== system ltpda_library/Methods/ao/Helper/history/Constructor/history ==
  Ground : Ground
  history : M-S-Function  Tag=history  FunctionName=ltpdasim
  Out1 : Outport  OutDataType=sfix(16)  OutScaling=2^0
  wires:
  Ground/1 -> history/1
  history/1 -> Out1/1

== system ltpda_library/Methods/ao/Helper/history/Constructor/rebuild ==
  Ground : Ground
  rebuild : M-S-Function  Tag=rebuild  FunctionName=ltpdasim
  Out1 : Outport  OutDataType=sfix(16)  OutScaling=2^0
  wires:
  Ground/1 -> rebuild/1
  rebuild/1 -> Out1/1

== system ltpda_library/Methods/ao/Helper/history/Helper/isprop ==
  In1 : Inport  OutDataType=sfix(16)  OutScaling=2^0
  isprop : M-S-Function  Tag=isprop  FunctionName=ltpdasim
  Out1 : Outport  OutDataType=sfix(16)  OutScaling=2^0
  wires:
  In1/1 -> isprop/1
  isprop/1 -> Out1/1

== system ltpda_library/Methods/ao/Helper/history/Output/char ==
  In1 : Inport  OutDataType=sfix(16)  OutScaling=2^0
  Terminator : Terminator
  char : M-S-Function  Tag=char  FunctionName=ltpdasim
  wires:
  char/1 -> Terminator/1
  In1/1 -> char/1

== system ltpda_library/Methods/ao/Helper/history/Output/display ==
  In1 : Inport  OutDataType=sfix(16)  OutScaling=2^0
  Terminator : Terminator
  display : M-S-Function  Tag=display  FunctionName=ltpdasim
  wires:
  display/1 -> Terminator/1
  In1/1 -> display/1

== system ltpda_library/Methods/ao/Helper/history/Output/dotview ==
  In1 : Inport  OutDataType=sfix(16)  OutScaling=2^0
  Terminator : Terminator
  dotview : M-S-Function  Tag=dotview  FunctionName=ltpdasim
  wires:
  dotview/1 -> Terminator/1
  In1/1 -> dotview/1

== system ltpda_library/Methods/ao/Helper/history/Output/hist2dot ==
  In1 : Inport  OutDataType=sfix(16)  OutScaling=2^0
  Terminator : Terminator
  hist2dot : M-S-Function  Tag=hist2dot  FunctionName=ltpdasim
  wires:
  hist2dot/1 -> Terminator/1
  In1/1 -> hist2dot/1

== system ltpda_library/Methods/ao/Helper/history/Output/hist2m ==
  In1 : Inport  OutDataType=sfix(16)  OutScaling=2^0
  Terminator : Terminator
  hist2m : M-S-Function  Tag=hist2m  FunctionName=ltpdasim
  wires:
  hist2m/1 -> Terminator/1
  In1/1 -> hist2m/1

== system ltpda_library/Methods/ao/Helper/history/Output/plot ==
  In1 : Inport  OutDataType=sfix(16)  OutScaling=2^0
  Terminator : Terminator
  plot : M-S-Function  Tag=plot  FunctionName=ltpdasim
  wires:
  plot/1 -> Terminator/1
  In1/1 -> plot/1

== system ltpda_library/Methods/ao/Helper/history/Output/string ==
  In1 : Inport  OutDataType=sfix(16)  OutScaling=2^0
  Terminator : Terminator
  string : M-S-Function  Tag=string  FunctionName=ltpdasim
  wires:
  string/1 -> Terminator/1
  In1/1 -> string/1

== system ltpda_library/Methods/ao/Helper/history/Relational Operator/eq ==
  In1 : Inport  OutDataType=sfix(16)  OutScaling=2^0
  eq : M-S-Function  Tag=eq  FunctionName=ltpdasim
  Out1 : Outport  OutDataType=sfix(16)  OutScaling=2^0
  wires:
  In1/1 -> eq/1
  eq/1 -> Out1/1

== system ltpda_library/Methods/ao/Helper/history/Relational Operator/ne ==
  In1 : Inport  OutDataType=sfix(16)  OutScaling=2^0
  ne : M-S-Function  Tag=ne  FunctionName=ltpdasim
  Out1 : Outport  OutDataType=sfix(16)  OutScaling=2^0
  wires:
  In1/1 -> ne/1
  ne/1 -> Out1/1

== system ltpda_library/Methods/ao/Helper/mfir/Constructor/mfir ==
  Ground : Ground
  mfir : M-S-Function  Tag=mfir  FunctionName=ltpdasim
  Out1 : Outport  OutDataType=sfix(16)  OutScaling=2^0
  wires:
  Ground/1 -> mfir/1
  mfir/1 -> Out1/1

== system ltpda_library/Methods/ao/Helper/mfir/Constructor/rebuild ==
  Ground : Ground
  rebuild : M-S-Function  Tag=rebuild  FunctionName=ltpdasim
  Out1 : Outport  OutDataType=sfix(16)  OutScaling=2^0
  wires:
  Ground/1 -> rebuild/1
  rebuild/1 -> Out1/1

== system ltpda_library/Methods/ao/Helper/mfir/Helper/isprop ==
  In1 : Inport  OutDataType=sfix(16)  OutScaling=2^0
  isprop : M-S-Function  Tag=isprop  FunctionName=ltpdasim
  Out1 : Outport  OutDataType=sfix(16)  OutScaling=2^0
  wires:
  In1/1 -> isprop/1
  isprop/1 -> Out1/1

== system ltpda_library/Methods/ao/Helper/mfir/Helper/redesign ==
  In1 : Inport  OutDataType=sfix(16)  OutScaling=2^0
  redesign : M-S-Function  Tag=redesign  FunctionName=ltpdasim
  Out1 : Outport  OutDataType=sfix(16)  OutScaling=2^0
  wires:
  In1/1 -> redesign/1
  redesign/1 -> Out1/1

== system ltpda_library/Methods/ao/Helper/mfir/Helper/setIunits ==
  In1 : Inport  OutDataType=sfix(16)  OutScaling=2^0
  setIunits : M-S-Function  Tag=setIunits  FunctionName=ltpdasim
  Out1 : Outport  OutDataType=sfix(16)  OutScaling=2^0
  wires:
  In1/1 -> setIunits/1
  setIunits/1 -> Out1/1

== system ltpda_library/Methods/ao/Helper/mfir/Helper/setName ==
  In1 : Inport  OutDataType=sfix(16)  OutScaling=2^0
  setName : M-S-Function  Tag=setName  FunctionName=ltpdasim
  Out1 : Outport  OutDataType=sfix(16)  OutScaling=2^0
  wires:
  In1/1 -> setName/1
  setName/1 -> Out1/1

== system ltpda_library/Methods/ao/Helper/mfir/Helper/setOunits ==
  In1 : Inport  OutDataType=sfix(16)  OutScaling=2^0
  setOunits : M-S-Function  Tag=setOunits  FunctionName=ltpdasim
  Out1 : Outport  OutDataType=sfix(16)  OutScaling=2^0
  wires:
  In1/1 -> setOunits/1
  setOunits/1 -> Out1/1

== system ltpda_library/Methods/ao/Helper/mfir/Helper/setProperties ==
  In1 : Inport  OutDataType=sfix(16)  OutScaling=2^0
  setProperties : M-S-Function  Tag=setProperties  FunctionName=ltpdasim
  Out1 : Outport  OutDataType=sfix(16)  OutScaling=2^0
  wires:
  In1/1 -> setProperties/1
  setProperties/1 -> Out1/1

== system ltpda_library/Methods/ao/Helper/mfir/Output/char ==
  In1 : Inport  OutDataType=sfix(16)  OutScaling=2^0
  Terminator : Terminator
  char : M-S-Function  Tag=char  FunctionName=ltpdasim
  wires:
  char/1 -> Terminator/1
  In1/1 -> char/1

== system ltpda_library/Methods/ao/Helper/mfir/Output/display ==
  In1 : Inport  OutDataType=sfix(16)  OutScaling=2^0
  Terminator : Terminator
  display : M-S-Function  Tag=display  FunctionName=ltpdasim
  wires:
  display/1 -> Terminator/1
  In1/1 -> display/1

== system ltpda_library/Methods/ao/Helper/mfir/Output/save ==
  In1 : Inport  OutDataType=sfix(16)  OutScaling=2^0
  Terminator : Terminator
  report : M-S-Function  Tag=report  FunctionName=ltpdasim
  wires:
  report/1 -> Terminator/1
  In1/1 -> report/1

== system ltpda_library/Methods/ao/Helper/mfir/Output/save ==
  In1 : Inport  OutDataType=sfix(16)  OutScaling=2^0
  Terminator : Terminator
  save : M-S-Function  Tag=save  FunctionName=ltpdasim
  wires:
  save/1 -> Terminator/1
  In1/1 -> save/1

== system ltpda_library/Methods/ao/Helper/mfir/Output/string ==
  In1 : Inport  OutDataType=sfix(16)  OutScaling=2^0
  Terminator : Terminator
  string : M-S-Function  Tag=string  FunctionName=ltpdasim
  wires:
  string/1 -> Terminator/1
  In1/1 -> string/1

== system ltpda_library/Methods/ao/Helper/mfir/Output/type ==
  In1 : Inport  OutDataType=sfix(16)  OutScaling=2^0
  Terminator : Terminator
  type : M-S-Function  Tag=type  FunctionName=ltpdasim
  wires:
  type/1 -> Terminator/1
  In1/1 -> type/1

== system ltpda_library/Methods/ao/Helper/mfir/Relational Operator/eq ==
  In1 : Inport  OutDataType=sfix(16)  OutScaling=2^0
  eq : M-S-Function  Tag=eq  FunctionName=ltpdasim
  Out1 : Outport  OutDataType=sfix(16)  OutScaling=2^0
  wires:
  In1/1 -> eq/1
  eq/1 -> Out1/1

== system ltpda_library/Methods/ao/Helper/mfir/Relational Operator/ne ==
  In1 : Inport  OutDataType=sfix(16)  OutScaling=2^0
  ne : M-S-Function  Tag=ne  FunctionName=ltpdasim
  Out1 : Outport  OutDataType=sfix(16)  OutScaling=2^0
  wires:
  In1/1 -> ne/1
  ne/1 -> Out1/1

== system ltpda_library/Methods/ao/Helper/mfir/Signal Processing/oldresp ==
  In1 : Inport  OutDataType=sfix(16)  OutScaling=2^0
  oldresp : M-S-Function  Tag=oldresp  FunctionName=ltpdasim
  Out1 : Outport  OutDataType=sfix(16)  OutScaling=2^0
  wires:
  In1/1 -> oldresp/1
  oldresp/1 -> Out1/1

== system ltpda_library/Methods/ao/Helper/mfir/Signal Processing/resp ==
  In1 : Inport  OutDataType=sfix(16)  OutScaling=2^0
  resp : M-S-Function  Tag=resp  FunctionName=ltpdasim
  Out1 : Outport  OutDataType=sfix(16)  OutScaling=2^0
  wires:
  In1/1 -> resp/1
  resp/1 -> Out1/1

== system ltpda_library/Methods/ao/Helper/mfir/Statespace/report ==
  In1 : Inport  OutDataType=sfix(16)  OutScaling=2^0
  report : M-S-Function  Tag=report  FunctionName=ltpdasim
  Out1 : Outport  OutDataType=sfix(16)  OutScaling=2^0
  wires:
  In1/1 -> report/1
  report/1 -> Out1/1

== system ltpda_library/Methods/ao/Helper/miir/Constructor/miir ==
  Ground : Ground
  miir : M-S-Function  Tag=miir  FunctionName=ltpdasim
  Out1 : Outport  OutDataType=sfix(16)  OutScaling=2^0
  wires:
  Ground/1 -> miir/1
  miir/1 -> Out1/1

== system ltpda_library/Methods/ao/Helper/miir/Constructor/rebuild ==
  Ground : Ground
  rebuild : M-S-Function  Tag=rebuild  FunctionName=ltpdasim
  Out1 : Outport  OutDataType=sfix(16)  OutScaling=2^0
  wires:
  Ground/1 -> rebuild/1
  rebuild/1 -> Out1/1
